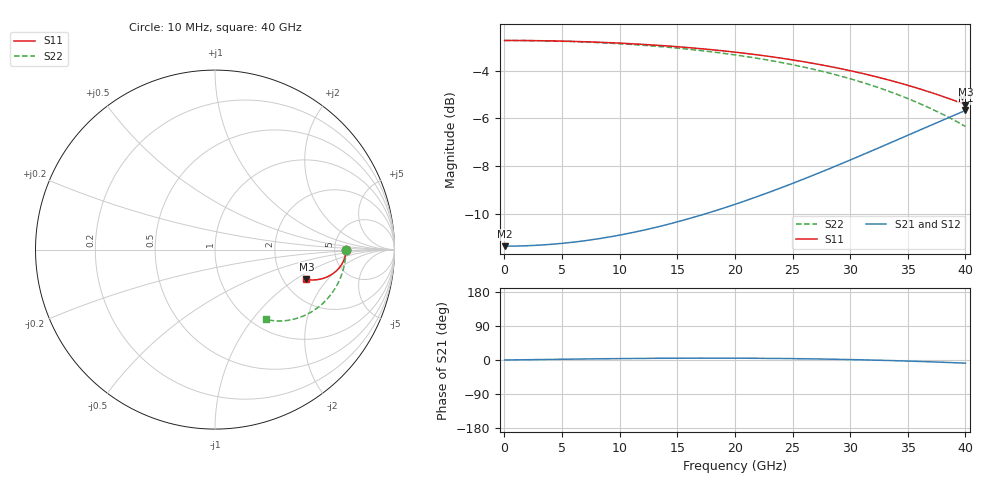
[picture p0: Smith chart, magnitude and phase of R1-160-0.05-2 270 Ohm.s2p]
!version-1
!date-03.2021
# MHz S RI R 50
!Freq ReS11 ImS11 ReS21 ImS21 ReS12 ImS12 ReS22 ImS22
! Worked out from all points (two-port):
!   801 points, 10 MHz to 40 GHz, reference 50 ohm
!   highest |S21| = -5.67 dB at 40 GHz (marker M1); lowest = -11.4 dB at 10 MHz (marker M2)
!   |S21| within 3 dB of the highest: 25.32 GHz to end of sweep
!   lowest |S11| = -5.4 dB at 40 GHz (marker M3), VSWR 3.30, Z = 133 - j61.9 ohm
!   |S11| at or under -10 dB: nowhere
!   |S22| runs from -6.3 to -2.7 dB; largest |S21 - S12| = 0
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10  0.7297 -5.92e-05  0.2703 1.99e-05  0.2703 1.99e-05  0.7297 -0.000148
3360  0.7284 -0.0199  0.2719 0.00664  0.2719 0.00664  0.7268 -0.0495
6710  0.7245 -0.0396  0.2766 0.013  0.2766 0.013  0.7179 -0.0986
10060  0.7178 -0.0592  0.2847 0.0187  0.2847 0.0187  0.703 -0.1469
13360  0.7084 -0.0782  0.296 0.0234  0.296 0.0234  0.6821 -0.1932
15060  0.7024 -0.0878  0.3032 0.0252  0.3032 0.0252  0.6688 -0.2164
16710  0.6958 -0.0969  0.311 0.0266  0.311 0.0266  0.6543 -0.2384
18360  0.6884 -0.1059  0.3199 0.0275  0.3199 0.0275  0.6381 -0.2597
20010  0.6801 -0.1146  0.3296 0.0277  0.3296 0.0277  0.6203 -0.2801
21710  0.6707 -0.1232  0.3407 0.0272  0.3407 0.0272  0.6 -0.3002
23360  0.6607 -0.1312  0.3525 0.0258  0.3525 0.0258  0.5786 -0.3186
25010  0.6497 -0.1387  0.3653 0.0234  0.3653 0.0234  0.5555 -0.3356
26710  0.6374 -0.1459  0.3794 0.0198  0.3794 0.0198  0.5299 -0.3515
28460  0.6236 -0.1525  0.395 0.0146  0.395 0.0146  0.5017 -0.3659
30160  0.6093 -0.1581  0.4111 0.00781  0.4111 0.00781  0.4726 -0.3777
31810  0.5944 -0.1626  0.4276 -0.000509  0.4276 -0.000509  0.443 -0.3868
33360  0.5795 -0.1659  0.4436 -0.0101  0.4436 -0.0101  0.4141 -0.3931
35060  0.5625 -0.1683  0.4617 -0.0228  0.4617 -0.0228  0.3814 -0.397
36710  0.5451 -0.1692  0.4796 -0.0376  0.4796 -0.0376  0.349 -0.3977
38310  0.5277 -0.1687  0.497 -0.0544  0.497 -0.0544  0.3174 -0.3952
39810  0.511 -0.1668  0.513 -0.0725  0.513 -0.0725  0.2879 -0.39
40000  0.5088 -0.1665  0.515 -0.075  0.515 -0.075  0.2842 -0.3891
